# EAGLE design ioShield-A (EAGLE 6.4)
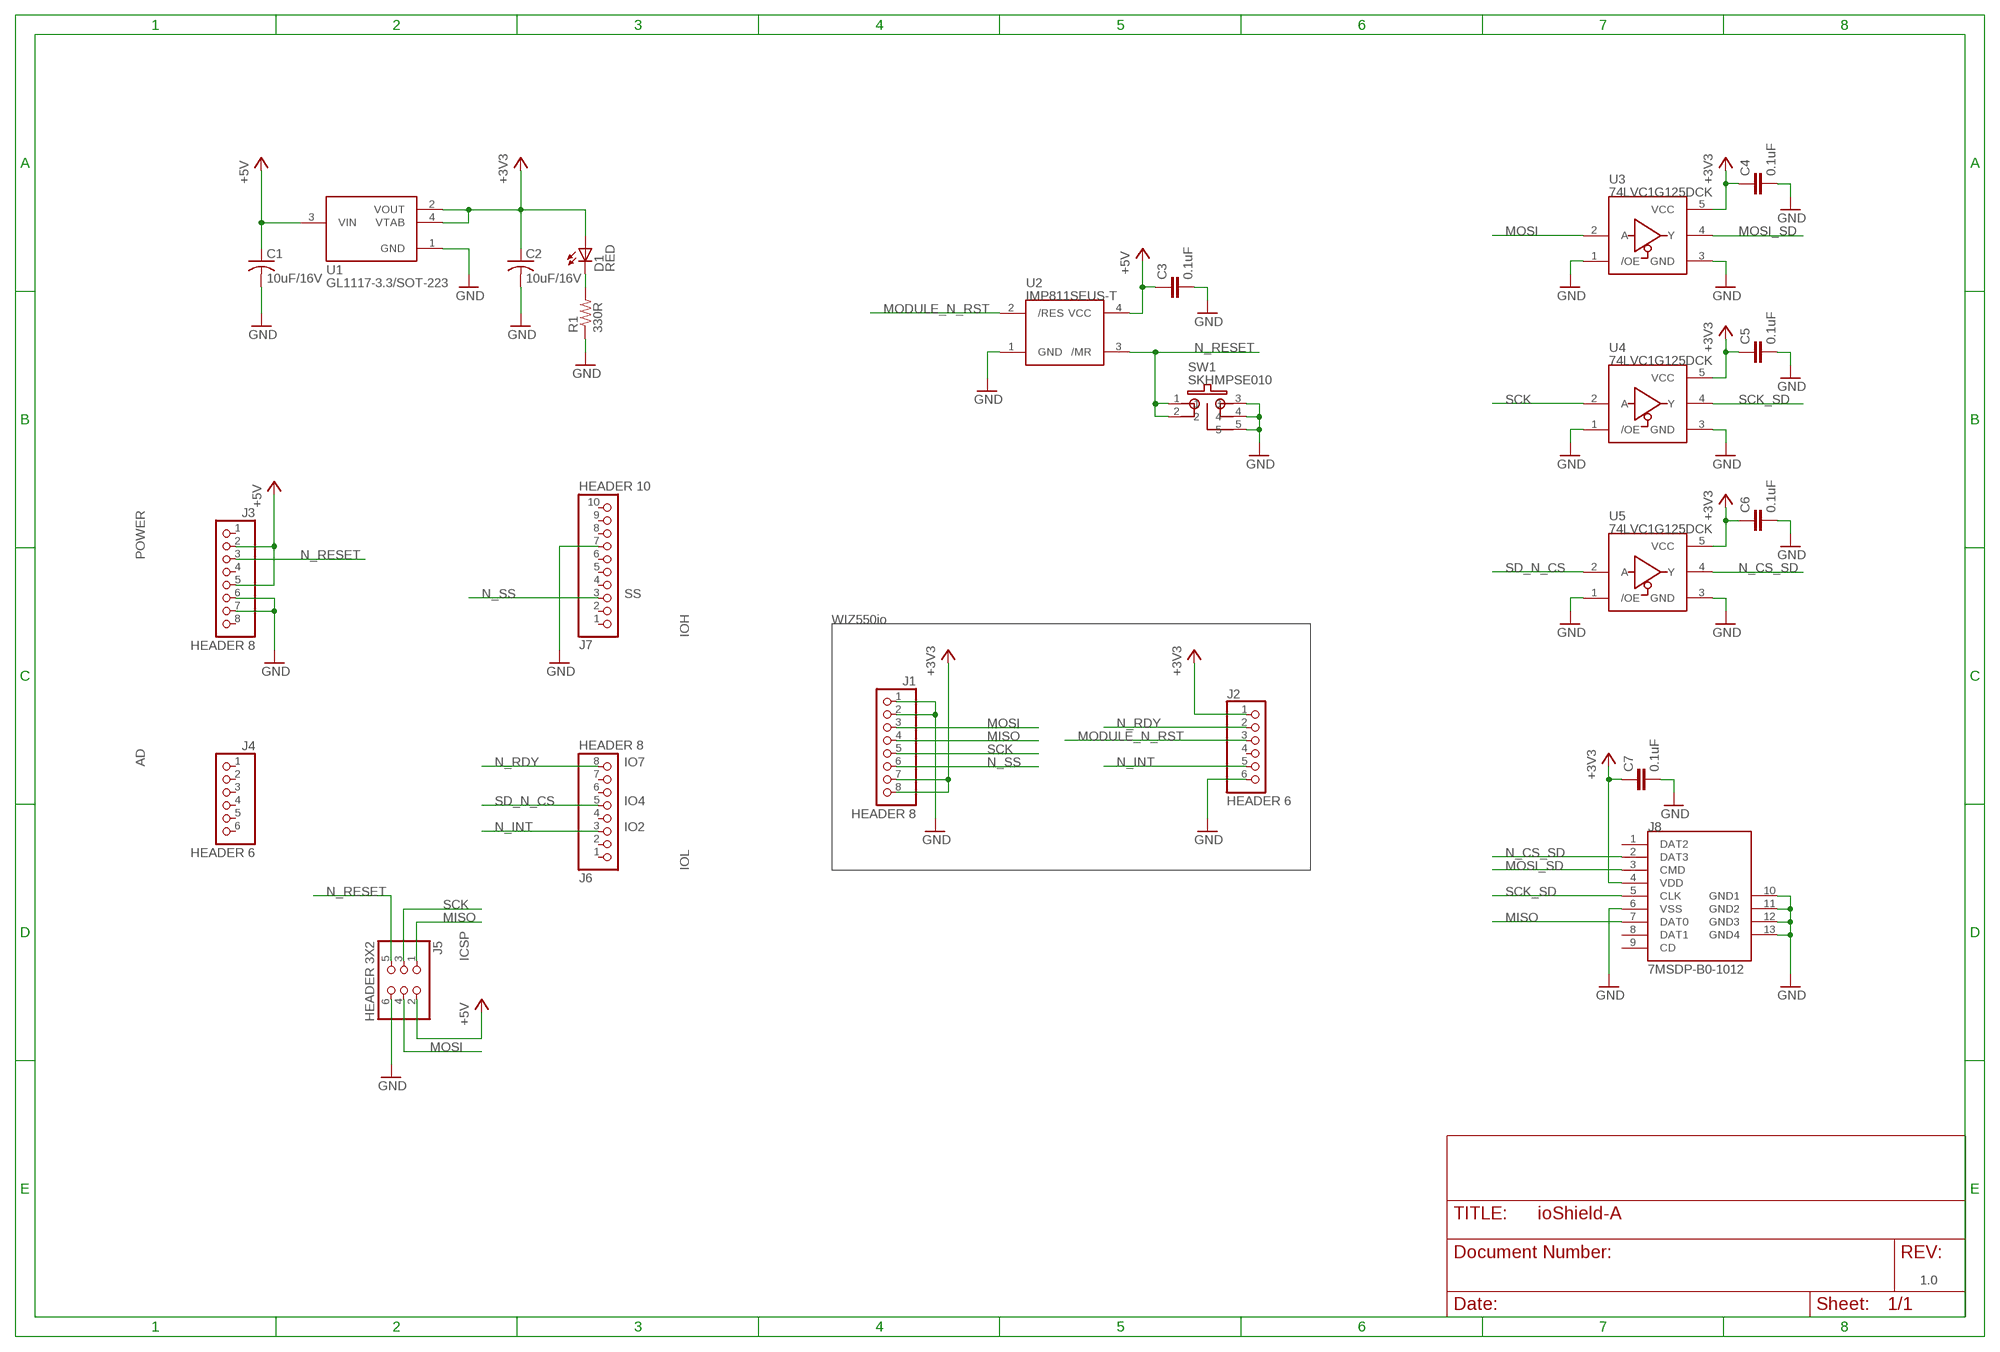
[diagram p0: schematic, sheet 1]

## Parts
C1  10uF/16V  CT-A(3216)  [CT-A(3216)]
C2  10uF/16V  CT-A(3216)  [CT-A(3216)]
C3  0.1uF  C1608  [C1608]
C4  0.1uF  C1608  [C1608]
C5  0.1uF  C1608  [C1608]
C6  0.1uF  C1608  [C1608]
C7  0.1uF  C1608  [C1608]
D1  RED  LED1608  [CHIP-LED1608]
J1  HEADER 8  HEADER8  [HEADER1X8]
J2  HEADER 6  HEADER6  [HEADER1X6]
J3  HEADER 8  HEADER8  [HEADER1X8]
J4  HEADER 6  HEADER6  [HEADER1X6]
J5  HEADER 3X2  HEADER3X2  [HEADER3X2]
J6  HEADER 8  HEADER8  [HEADER1X8]
J7  HEADER 10  HEADER10  [HEADER1X10]
J8  7MSDP-B0-1012  [MICROSD_HC]
R1  330R  R1608  [R1608]
SW1  SKHMPSE010  TACT_6.2X6.5  [TACT_6.2X6.5]
U1  GL1117-3.3/SOT-223  [SOT223_HC]
U2  IMP811SEUS-T  [SOT-143]
U3  74LVC1G125DCK  SN74LVC1G125  [SC70-5(DCK)]
U4  74LVC1G125DCK  SN74LVC1G125  [SC70-5(DCK)]
U5  74LVC1G125DCK  SN74LVC1G125  [SC70-5(DCK)]

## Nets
+3V3: C2.+ C4.1 C5.1 C6.1 C7.1 D1.A J1.7 J1.8 J2.1 J8.4(VDD) U1.2(VOUT) U1.4(VTAB) U3.5(VCC) U4.5(VCC) U5.5(VCC)
+5V: C1.+ C3.1 J3.2 J3.5 J5.2 U1.3(VIN) U2.4(VCC)
GND: C1.- C2.- C3.2 C4.2 C5.2 C6.2 C7.2 J1.1 J1.2 J2.6 J3.6 J3.7 J5.6 J7.7 J8.6(VSS) J8.10(GND1) J8.11(GND2) J8.12(GND3) J8.13(GND4) R1.1 SW1.3 SW1.4 SW1.5 U1.1(GND) U2.1(GND) U3.1(/OE) U3.3(GND) U4.1(/OE) U4.3(GND) U5.1(/OE) U5.3(GND)
MISO: J1.4 J5.1 J8.7(DAT0)
MODULE_N_RST: J2.3 U2.2(/RES)
MOSI: J1.3 J5.4 U3.2(A)
MOSI_SD: J8.3(CMD) U3.4(Y)
N$1: D1.C R1.2
N_CS_SD: J8.2(DAT3) U5.4(Y)
N_INT: J2.5 J6.3
N_RDY: J2.2 J6.8
N_RESET: J3.3 J5.5 SW1.1 SW1.2 U2.3(/MR)
N_SS: J1.6 J7.3
SCK: J1.5 J5.3 U4.2(A)
SCK_SD: J8.5(CLK) U4.4(Y)
SD_N_CS: J6.5 U5.2(A)
Unconnected: J2.4 J3.1 J3.4 J3.8 J4.1 J4.2 J4.3 J4.4 J4.5 J4.6 J6.1 J6.2 J6.4 J6.6 J6.7 J7.1 J7.2 J7.4 J7.5 J7.6 J7.8 J7.9 J7.10 J8.1(DAT2) J8.8(DAT1) J8.9(CD)

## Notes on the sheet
- POWER
- SS
- WIZ550io
- IOH
- AD | IO7
- IO4
- IO2
- IOL
- ICSP
- 1.0

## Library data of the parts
C1 C2 = rlc_HC:CT-A(3216): CT-A(3216)
C3-C7 = rlc_HC:C1608: C1608
D1 = rlc_HC:LED1608: LED 1608
J1 J3 J6 = pinheader_HC:HEADER8: HEADER 1X8 2.54mm
J2 J4 = pinheader_HC:HEADER6: HEADER 1X6 2.54mm
J5 = pinheader_HC:HEADER3X2: HEADER 3X2 2.54mm
J7 = pinheader_HC:HEADER10: HEADER 1X10 2.54mm
J8 = socket_HC:7MSDP-B0-1012: Micro SD Connector Part No. 7MSDP-B0-1012
R1 = rlc_HC:R1608: R1608
SW1 = switch_HC:TACT_6.2X6.5: ALPS TACT_6.2X6.5
U1 = dc-dc:GL1117-3.3/SOT-223: GL1117-3.3/SOT-223
U2 = jjam_HC:IMP811SEUS-T: IMP811SEUS-T SOT-143
U3-U5 = jjam_HC:SN74LVC1G125: SN74LVC1G125 DCK(SC70)

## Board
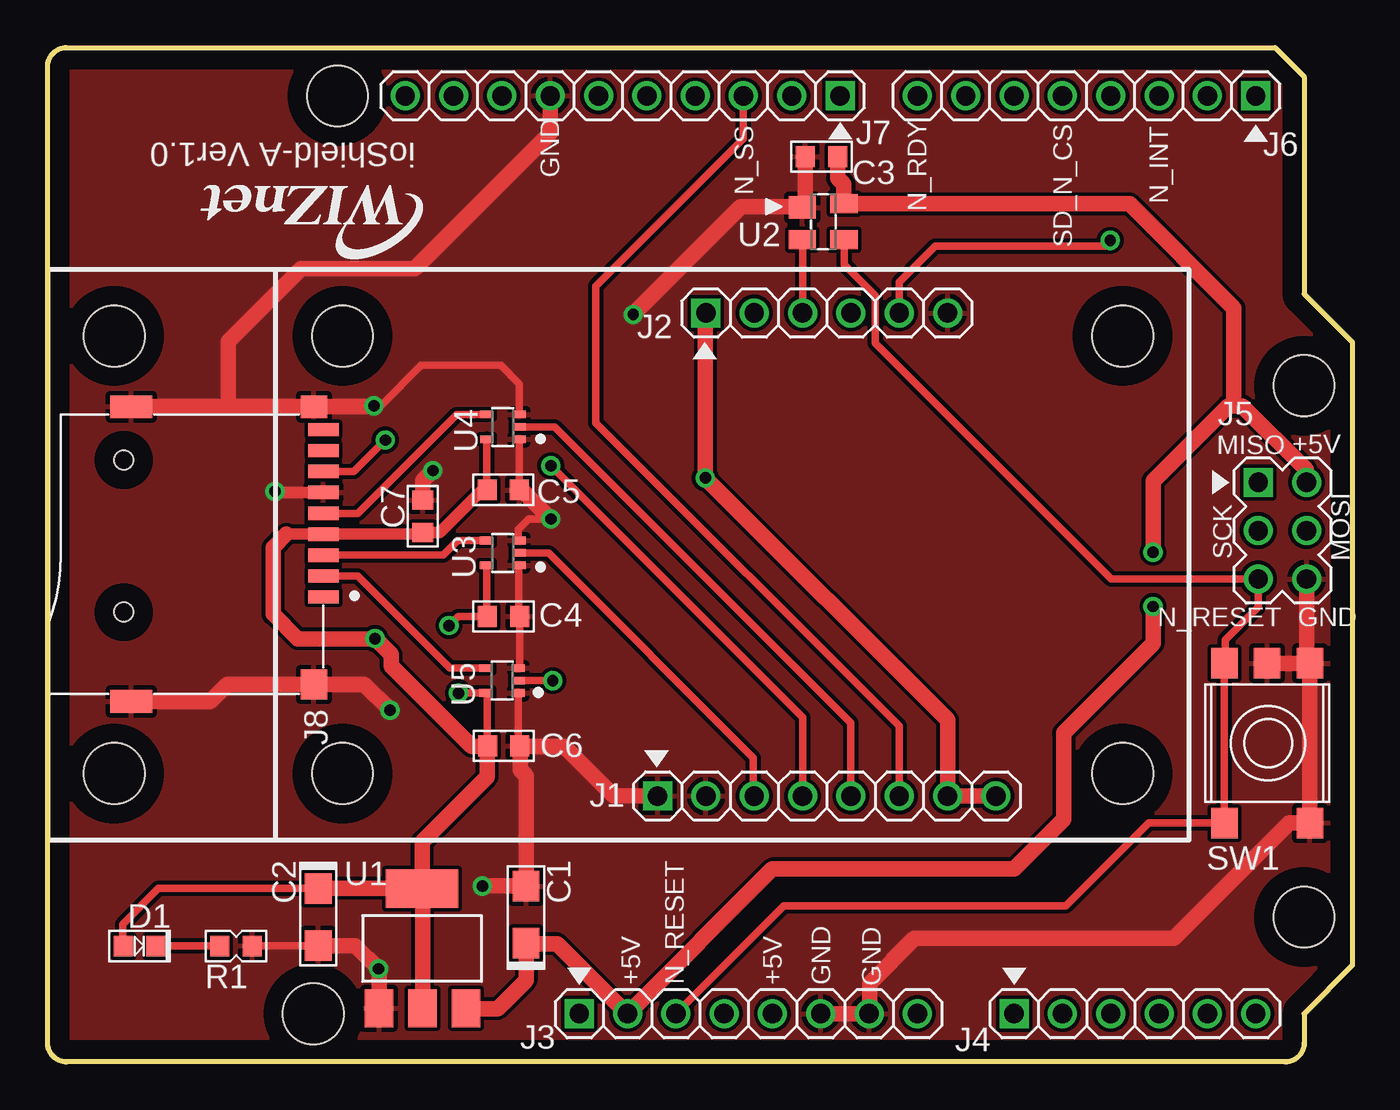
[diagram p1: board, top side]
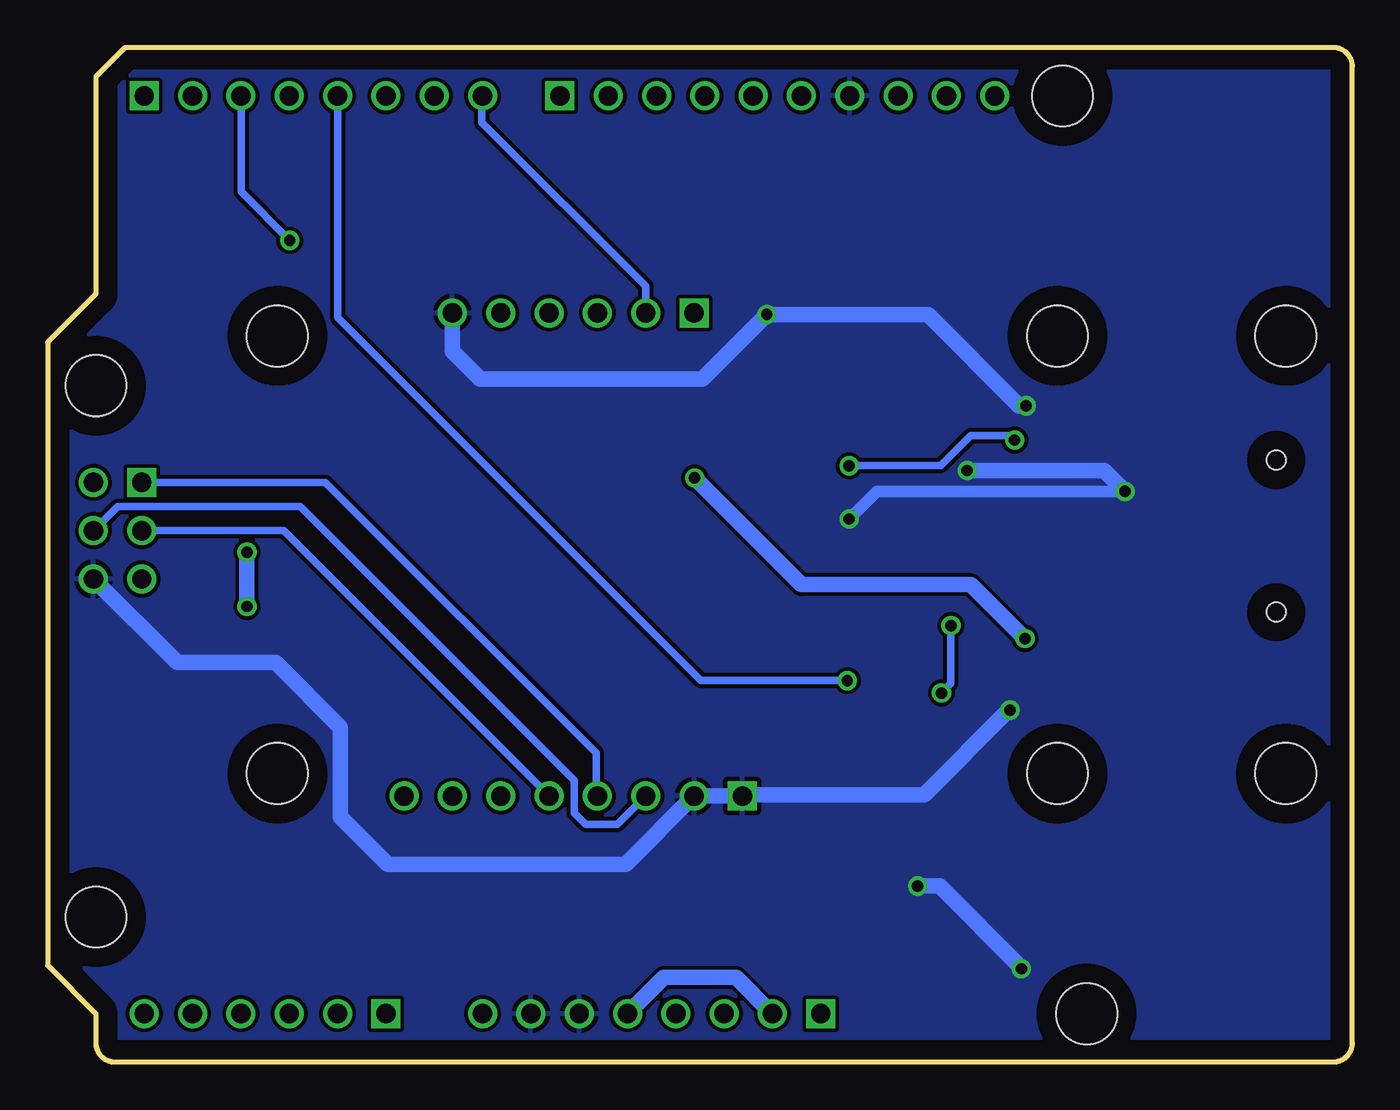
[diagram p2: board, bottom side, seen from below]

Size 68.58 x 53.34 mm. Coordinates in mm from the lower left corner, seen from the top.
Outline: 64.52,53.34 66.04,51.82 66.04,40.39 68.58,37.85 68.58,5.08 66.04,2.54 66.04,1 arc-90 65.04,0 1,0 arc-90 0,1 0,52.34 arc-90 1,53.34 64.52,53.34
Copper layers (1*16): Top 0.035mm / dielectric 1.5mm / Bottom 0.035mm
Design rules "default *": minimum track width 10mil, minimum drill 23mil, track to track 8mil, track to pad 8mil, pad to pad 8mil, via to via 8mil, smd to smd 8mil, copper to edge 40mil, drill to drill 8mil, minimum pad ring 10mil, minimum via ring 8mil, stop-mask expansion 4mil, vias tented up to drill 0mil, thermal gap 10mil
Holes 3.2 mm at 15.24,50.8 13.97,2.54 66.04,35.56 66.04,7.62 3.5,15.17 3.5,38.17 56.5,15.17 56.5,38.17 15.5,15.17 15.5,38.17

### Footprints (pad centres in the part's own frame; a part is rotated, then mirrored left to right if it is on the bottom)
CT-A(3216) = smd 1.6 x 1.4: + -1.5,0; - 1.5,0
C1608 = smd 1 x 1.1: 1 -0.85,0; 2 0.85,0
CHIP-LED1608 = smd 1 x 1.1: A -0.85,0; C 0.85,0
HEADER1X8 = drill 1.016 square: 1 -8.89,0 | drill 1.016: 2 -6.35,0; 3 -3.81,0; 4 -1.27,0; 5 1.27,0; 6 3.81,0; 7 6.35,0; 8 8.89,0
HEADER1X6 = drill 1.016 square: 1 -6.35,0 | drill 1.016: 2 -3.81,0; 3 -1.27,0; 4 1.27,0; 5 3.81,0; 6 6.35,0
HEADER3X2 = drill 1.016 square: 1 0,0 | drill 1.016: 2 0,-2.54; 3 -2.54,0; 4 -2.54,-2.54; 5 -5.08,0; 6 -5.08,-2.54
HEADER1X10 = drill 1.016 square: 1 -11.43,0 | drill 1.016: 2 -8.89,0; 3 -6.35,0; 4 -3.81,0; 5 -1.27,0; 6 1.27,0; 7 3.81,0; 8 6.35,0; 9 8.89,0; 10 11.43,0
MICROSD_HC = smd 0.7 x 1.6: 1 10.6,11.2; 2 9.5,11.2; 3 8.4,11.2; 4 7.3,11.2; 5 6.2,11.2; 6 5.1,11.2; 7 4,11.2; 8 2.9,11.2; 9 1.8,11.2 | smd 1.2 x 1.4: 10 0.6,10.7 | smd 1.6 x 1.4: 11 15.2,10.7 | smd 1.2 x 2.2: 12 16.1,1.1; 13 0.6,1.1 | hole 1: 3.4,0.7; 11.4,0.7
R1608 = smd 1 x 1.1: 1 -0.85,0; 2 0.85,0
TACT_6.2X6.5 = smd 1.6 x 1.4: 1 -4.2,0; 2 4.2,0; 3 -4.2,-4.5; 4 4.2,-4.5; 5 4.2,-2.25
SOT223_HC = smd 1.499 x 2.007: 1 -2.261,-3.15; 2 0.025,-3.15; 3 2.311,-3.15 | smd 3.81 x 2.007: 4 0,3.15
SOT-143 = smd 1.2 x 1.44: 1 -0.75,-1.1 | smd 1 x 1.44: 2 0.95,-1.1; 3 0.95,1.1; 4 -0.95,1.1
SC70-5(DCK) = smd 0.4 x 0.7: 1 -0.65,-0.85; 2 0,-0.85; 3 0.65,-0.85; 4 0.65,0.85; 5 -0.65,0.85

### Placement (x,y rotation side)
C1  25.15,7.75 90 top
C2  14.22,7.62 270 top
C3  40.68,47.6 180 top
C4  23.96,23.43 0 top
C5  23.95,30.09 0 top
C6  23.98,16.62 0 top
C7  19.72,28.7 90 top
D1  4.83,6.1 0 top
J1  40.95,13.98 0 top
J2  40.95,39.38 0 top
J3  36.83,2.54 0 top
J4  57.15,2.54 0 top
J5  63.63,30.48 90 top
J6  54.61,50.8 180 top
J7  30.23,50.8 180 top
J8  3.3,35.05 270 top
R1  9.91,6.1 180 top
SW1  61.85,16.76 90 top
U1  19.68,5.97 0 top
U2  40.76,44.18 270 top
U3  23.92,26.77 90 top
U4  23.93,33.4 90 top
U5  23.89,20.06 90 top

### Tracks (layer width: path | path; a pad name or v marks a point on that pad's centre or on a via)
+3V3  (via drill 0.6)
  Top 0.406: C2.+ 5.82,9.12 3.95,7.25 3.95,6.12 D1.A | U4.5 23.08,30.1 C5.1 | U3.5 23.07,23.47 C4.1 21.58,23.43 v21.1,22.95 | v21.6,19.4 U5.5 23.1,19.35 23.1,16.65
  Top 0.61: C5.1 22.84,30.09 20.6,27.85 C7.1 19.62,27.75 J8.4 12.55,27.75
  Top 0.813: U1.2 19.71,9.09 U1.4 | U1.4 C2.+ | 23.1,16.65 C6.1 23.1,16.6 | U1.4 19.68,11.59 23.1,15 23.1,16.6 | 12.55,27.75 11.85,27.05 11.85,23.55 13.15,22.25 v17.2,22.25 v17.21,22.26 18.05,21.42 18.05,20.83 22.28,16.6 23.1,16.6 | J1.8 J1.7 47.3,17.98 v34.57,30.71 34.57,39.35 J2.1
  Bottom 0.406: v21.1,22.95 21.1,19.9 v21.6,19.4
  Bottom 0.813: v17.21,22.26 17.23,22.26 20.07,25.1 28.96,25.1 v34.57,30.71
+5V  (via drill 0.6)
  Top 0.813: C1.+ | C1.+ 25.15,4.3 23.65,2.8 22.02,2.8 U1.3 | C3.1 41.53,46.47 41.85,46.15 41.85,45.15 U2.4 56.87,45.13 62.35,39.65 62.35,34.55 62.4,34.5 | J5.2 66.15,30.5 66.15,31.15 62.8,34.5 62.4,34.5 | v58.1,23.95 58.1,22 53.4,17.3 53.4,12.75 50.8,10.15 38.09,10.15 J3.2 30.46,2.54 26.8,6.2 25.19,6.2 C1.+ | 62.4,34.5 62.05,34.5 58.1,30.55 v58.1,26.8
  Bottom 0.813: v58.1,26.8 v58.1,23.95 | J3.5 36.2,4.45 32.39,4.45 J3.2
GND  (via drill 0.6)
  Top 0.406: R1.1 14.2,6.1 C2.- | v26.45,28.55 25.3,28.55 24.75,28 24.75,27.44 U3.3 | U5.3 24.81,20.78 C4.2 24.77,23.47 U3.1 | U5.1 24.74,16.71 C6.2 | C5.2 24.8,32.73 U4.1 | U4.3 24.8,34.06 24.8,35.65 23.81,36.64 19.64,36.64 17.5,34.5 v17.15,34.5
  Top 0.61: J8.6 12,29.95 v11.95,30
  Top 0.813: U1.1 17.42,4.88 v17.4,4.9 16.18,6.12 C2.- | v22.85,9.25 C1.- 25.15,15.05 24.85,15.35 24.85,16.6 | J5.6 66.17,21.15 SW1.4 | SW1.5 SW1.4 | SW1.4 SW1.3 65.26,12.56 59.2,6.5 45.55,6.5 43.2,4.15 43.2,2.56 J3.7 J3.6 | 39.65,44.95 U2.1 | C3.2 39.83,45.1 U2.1 | J1.1 29.77,13.98 27.15,16.6 24.85,16.6 | 24.85,16.6 C6.2 | C7.2 19.72,30.57 v20.25,31.1 | C5.2 24.91,30.09 v26.45,28.55 | J8.12 8.55,18.95 9.45,19.85 J8.11 16.65,19.85 v18,18.5 | J8.13 9.49,34.45 | 9.49,34.45 J8.10 17.1,34.45 v17.15,34.5 | v30.78,39.3 30.78,39.32 36.44,44.98 39.62,44.98 U2.1 | J7.7 26.43,50.79 26.43,48.84 19.3,41.71 13.33,41.71 9.49,37.87 9.49,34.45
  Bottom 0.61: v11.95,30 25,30 v26.45,28.55
  Bottom 0.813: v17.4,4.9 17.4,4.95 21.7,9.25 v22.85,9.25 | J5.6 61.77,21 56.6,21 53.2,17.6 53.2,12.9 50.7,10.4 38.2,10.4 34.62,13.98 J1.2 J1.1 32,14.05 22.5,14.05 18.05,18.5 v18,18.5 | v17.15,34.5 17.5,34.5 22.3,39.3 v30.78,39.3 34.17,35.91 45.84,35.91 47.3,37.37 J2.6 | v20.25,31.1 13.05,31.1 v11.95,30
  pour Top: 1.02,0 arc-90 0,1.02 0,52.32 arc-90 1.02,53.34 64.52,53.34 66.04,51.82 66.04,40.39 68.58,37.85 68.58,5.08 66.04,2.54 66.04,1.02 arc-90 65.02,0
  pour Bottom: 1.02,0 arc-90 0,1.02 0,52.32 arc-90 1.02,53.34 64.52,53.34 66.04,51.82 66.04,40.39 68.58,37.85 68.58,5.08 66.04,2.54 66.04,1.02 arc-90 65.02,0
MISO  (via drill 0.6)
  Top 0.406: J1.4 39.68,18.12 v26.45,31.35 | 14.55,31 J8.7 16.1,31.05 v17.75,32.7
  Bottom 0.406: J5.1 53.98,30.48 39.75,16.26 39.75,14.05 J1.4 | v26.45,31.35 21.65,31.35 20.05,32.95 18,32.95 v17.75,32.7
MODULE_N_RST
  Top 0.406: J2.3 39.68,43.22 U2.2
MOSI
  Top 0.406: U3.2 26.33,26.77 37.1,16 37.1,14.03 J1.3
  Bottom 0.406: J5.4 64.9,29.2 55.3,29.2 40.9,14.8 40.9,13.1 40.3,12.5 38.63,12.5 J1.3
MOSI_SD
  Top 0.406: U3.4 21.57,27.42 20.8,26.65 J8.3
N$1
  Top 0.406: D1.C R1.2
N_CS_SD
  Top 0.406: U5.4 21.14,20.71 16.3,25.55 J8.2
N_INT  (via drill 0.6)
  Top 0.406: J2.5 44.76,41.01 46.65,42.9 55.55,42.9 v55.85,43.2
  Bottom 0.406: v55.85,43.2 58.4,45.75 58.4,50.78 J6.3
N_RDY
  Bottom 0.406: J2.2 37.14,40.79 45.75,49.4 45.75,50.77 J6.8
N_RESET
  Top 0.406: 33.05,2.57 J3.3 38.68,8.2 53.5,8.2 57.86,12.56 SW1.1 SW1.2 61.9,21.02 61.9,22.2 63.63,23.93 J5.5 55.9,25.4 43.5,37.8 43.5,40.3 41.86,41.94 U2.3
N_SS
  Top 0.406: 44.75,14 J1.6 44.76,17.66 28.82,33.6 28.82,40.79 36.58,48.55 J7.3
SCK
  Top 0.406: 42.2,14.01 J1.5 42.22,17.15 42.22,17.52 42.22,17.83 26.66,33.39 U4.2
  Bottom 0.406: J5.3 56.18,27.94 J1.5
SCK_SD
  Top 0.406: U4.4 21.5,34.05 16.3,28.85 J8.5
SD_N_CS  (via drill 0.6)
  Top 0.406: v26.55,20.05 U5.2
  Bottom 0.406: J6.5 53.34,39.14 34.25,20.05 v26.55,20.05

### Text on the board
tPlace: ioShield-A Ver1.0 | GND | N_SS | N_RDY | N_INT | SD_N_CS | MISO | +5V | SCK | MOSI | N_RESET | GND | +5V | N_RESET | +5V | GND | GND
